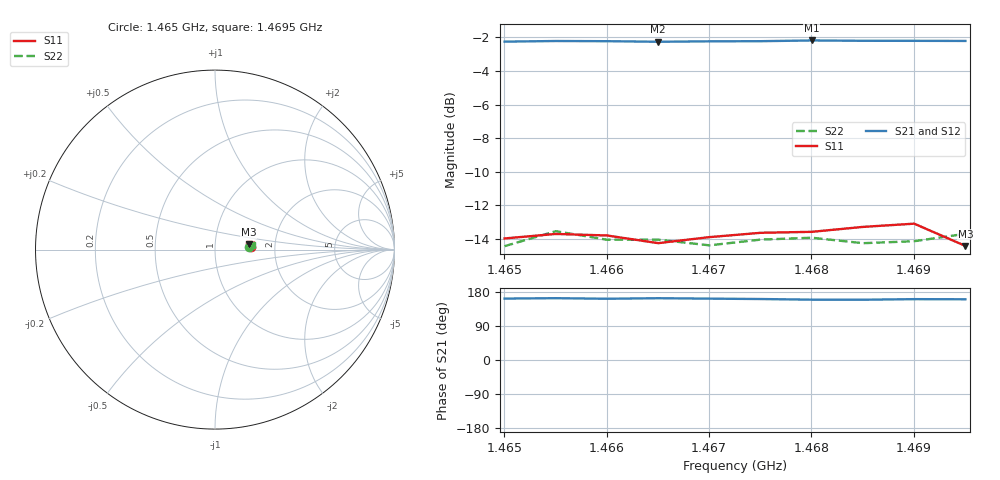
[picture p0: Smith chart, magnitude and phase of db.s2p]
#  HZ  S  DB  R  50
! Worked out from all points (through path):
!   10 points, 1.465 GHz to 1.4695 GHz, reference 50 ohm
!   highest |S21| = -2.19 dB at 1.468 GHz (marker M1); lowest = -2.3 dB at 1.4665 GHz (marker M2)
!   lowest |S11| = -14.4 dB at 1.4695 GHz (marker M3), VSWR 1.47, Z = 73 + j4.53 ohm
!   |S11| at or under -10 dB: start of sweep to end of sweep
!   |S22| runs from -14.4 to -13.5 dB; largest |S21 - S12| = 0.026
1.465004e9  -13.97 3.3  -2.26 162.1  -2.26 162.7  -14.43 4.5
1.465504e9  -13.70 3.5  -2.22 163.1  -2.23 161.2  -13.53 2.0
1.466004e9  -13.79 6.8  -2.23 161.6  -2.24 162.9  -14.04 2.5
1.466504e9  -14.25 4.7  -2.27 163.0  -2.28 163.8  -14.04 6.3
1.467004e9  -13.89 3.7  -2.24 161.9  -2.26 162.0  -14.38 4.4
1.467504e9  -13.63 4.5  -2.23 160.9  -2.23 162.1  -14.04 6.0
1.468005e9  -13.57 6.8  -2.19 159.2  -2.21 160.5  -13.92 5.8
1.468505e9  -13.28 4.3  -2.21 159.1  -2.21 157.5  -14.25 3.0
1.469005e9  -13.09 10.4  -2.21 160.6  -2.24 159.6  -14.13 7.3
1.469505e9  -14.41 9.0  -2.22 160.3  -2.26 160.3  -13.69 7.2
